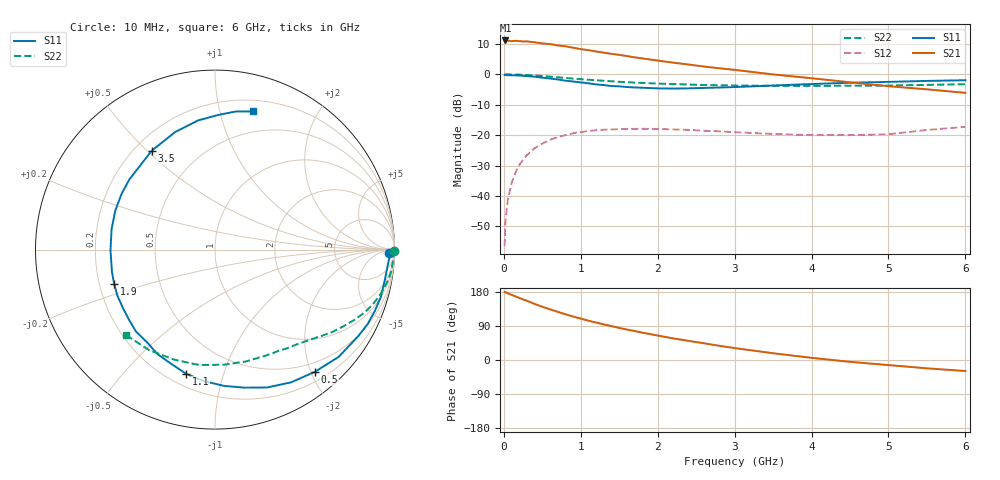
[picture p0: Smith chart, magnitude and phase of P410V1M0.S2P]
! SIEMENS Small Signal Semiconductors
! BFP182
! Si NPN RF Bipolar Junction Transistor in SOT143
! VCE = 10 V  IC = 1 mA
! Common Emitter S-Parameters:  March  1996
# GHz  S  MA  R  50
!  f  S11  S21  S12  S22
! GHz  MAG  ANG  MAG  ANG  MAG  ANG  MAG  ANG
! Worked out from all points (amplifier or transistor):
!   36 points, 10 MHz to 6 GHz, reference 50 ohm
!   highest |S21| = 11.1 dB at 20 MHz (marker M1)
!   |S21| within 3 dB of that: start of sweep to 1.045 GHz
!   unconditionally stable (mu >= 1): 2.654 GHz to end of sweep
!   at 250 MHz: K = 0.10, MSG = 19.4 dB, |S12| = -28.1 dB
!   at 1.4 GHz: K = 0.54, MSG = 12.4 dB, |S12| = -18.1 dB
!   at 6 GHz: K = 1.07, MAG = 4.0 dB, |S12| = -17.3 dB
!   S11 on the Smith chart (normalised r, x): 10 MHz: 51, -32; 500 MHz: 0.34, -2.06; 1.1 GHz: 0.27, -0.76; 1.9 GHz: 0.26, -0.16; 3.5 GHz: 0.27, +0.52; 6 GHz: 0.30, +1.27
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0.01  0.9721 -1.0  3.523 179.4  0.0015 87.7  0.9984 -0.3
0.02  0.9746 -2.0  3.596 178.9  0.0037 87.1  0.9952 -0.8
0.05  0.966 -5.3  3.564 176.1  0.0084 88.2  0.9962 -1.9
0.1  0.9614 -10.3  3.506 171.9  0.0161 82.2  0.9931 -3.8
0.15  0.9608 -16.0  3.548 167.9  0.0241 79.5  0.9903 -5.8
0.3  0.9329 -31.0  3.469 156.3  0.047 70.6  0.9728 -11.5
0.4  0.9122 -40.9  3.356 148.0  0.0609 64.7  0.9557 -14.9
0.5  0.8795 -50.7  3.215 140.5  0.0725 58.4  0.9361 -18.2
0.6  0.8526 -60.1  3.138 133.7  0.0839 53.3  0.9155 -21.2
0.8  0.7861 -78.1  2.884 120.7  0.1002 43.5  0.8709 -26.6
0.9  0.7607 -86.3  2.73 114.8  0.1073 39.1  0.8496 -28.9
1.1  0.71 -103.2  2.492 103.6  0.1169 31.4  0.8138 -33.1
1.3  0.6648 -118.7  2.266 93.9  0.1228 24.7  0.7821 -36.8
1.5  0.634 -134.0  2.085 84.6  0.1253 19.4  0.7525 -40.2
1.9  0.5935 -161.1  1.751 68.4  0.1269 10.5  0.7122 -46.4
2.2  0.5823 -179.6  1.553 57.2  0.1242 5.9  0.6897 -51.1
2.8  0.6063 149.1  1.256 37.5  0.1157 -0.1  0.6609 -61.0
3.5  0.6537 122.7  0.995 17.8  0.1047 -1.0  0.6466 -74.6
4  0.6918 108.7  0.861 5.8  0.1002 2.3  0.6434 -85.8
4.5  0.7261 97.4  0.739 -4.9  0.1003 6.0  0.6489 -98.0
5.5  0.7782 81.4  0.566 -22.0  0.1217 15.3  0.6696 -123.3
6  0.7985 74.5  0.496 -29.1  0.1367 14.7  0.6867 -135.9
